FUNCTION_BLOCK FB_Sample
VAR_INPUT
    bEnable : BOOL;
    nValue : INT;
END_VAR
VAR_OUTPUT
    bDone : BOOL;
    nResult : INT;
END_VAR
VAR
    _state : INT;
END_VAR

IF bEnable THEN
    _state := _state + 1;
    nResult := nValue * 2;
    bDone := TRUE;
ELSE
    bDone := FALSE;
END_IF

END_FUNCTION_BLOCK
